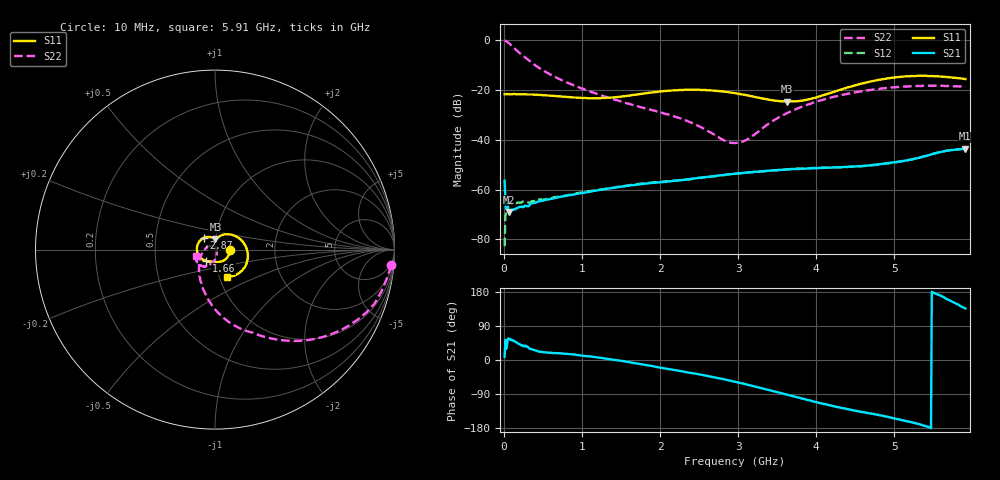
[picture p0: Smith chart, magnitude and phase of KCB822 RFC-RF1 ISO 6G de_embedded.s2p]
!Agilent	"Technologies,N5230A,MY45001650,A.07.50.48"
!Agilent	N5230A:	A.07.50.48
!Date:	"Wednesday,"	February	"12,"	2014	15:21:15
!Correction:	S11(Full	2	"Port(1,2))"
!S21(Full	2	"Port(1,2))"
!S12(Full	2	"Port(1,2))"
!S22(Full	2	"Port(1,2))"
!S2P	File:	Measurements:	"S11,"	"S21,"	"S12,"	S22:
#	Hz	S	dB	R	50
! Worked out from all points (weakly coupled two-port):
!   591 points, 10 MHz to 5.91 GHz, reference 50 ohm
!   highest |S21| = -43.60 dB at 5.9 GHz (marker M1); lowest = -69.0 dB at 60 MHz (marker M2)
!   lowest |S11| = -24.7 dB at 3.63 GHz (marker M3), VSWR 1.12, Z = 49.9 + j5.82 ohm
!   |S11| at or under -10 dB: start of sweep to end of sweep
!   |S22| runs from -41.3 to -0.1 dB; largest |S21 - S12| = 0.0016
!   S11 on the Smith chart (normalised r, x): 10 MHz: 1.18, -0.01; 1.66 GHz: 0.90, -0.12; 2.87 GHz: 0.87, +0.11; 5.91 GHz: 1.09, -0.34
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1e7  -21.70 -2.0  -56.40 8.3  -82.70 -164.0  -0.12 -5.2
4e7  -21.60 -3.9  -65.50 38.4  -65.30 10.4  -0.55 -18.8
6e7  -21.70 -5.3  -69.00 57.4  -63.80 34.0  -1.06 -26.2
8e7  -21.70 -6.9  -68.70 53.8  -65.20 115.0  -1.63 -33.0
1.1e8  -21.70 -9.6  -68.30 52.7  -65.80 -165.0  -2.53 -41.7
1.8e8  -21.70 -16.0  -67.30 44.1  -65.20 -85.6  -4.56 -57.1
3.5e8  -21.80 -31.9  -65.60 28.9  -64.90 27.8  -8.90 -86.2
5.6e8  -22.20 -51.2  -64.00 19.6  -63.70 21.6  -13.20 -109.0
1e9  -23.20 -85.9  -61.40 11.4  -61.10 13.1  -19.40 -143.0
1.66e9  -22.00 -127.0  -58.20 -7.6  -58.00 -8.0  -26.10 169.0
1.98e9  -20.70 -150.0  -57.10 -19.2  -56.90 -18.7  -28.80 147.0
2.38e9  -19.90 177.0  -55.80 -33.7  -55.80 -34.7  -32.90 121.0
2.87e9  -20.90 135.0  -53.90 -53.2  -53.90 -53.1  -40.80 52.1
2.96e9  -21.30 127.0  -53.60 -57.5  -53.70 -57.8  -41.30 27.7
3.13e9  -22.30 114.0  -53.10 -65.6  -53.10 -65.8  -39.60 -17.4
3.63e9  -24.70 87.7  -51.90 -91.7  -51.80 -91.7  -29.20 -74.8
3.95e9  -23.40 77.6  -51.40 -109.0  -51.30 -109.0  -25.20 -89.3
4.38e9  -19.20 51.5  -50.90 -129.0  -50.90 -129.0  -21.70 -104.0
4.93e9  -15.30 5.7  -49.30 -151.0  -49.40 -151.0  -19.10 -122.0
5.39e9  -14.30 -31.4  -46.60 -174.0  -46.60 -173.0  -18.30 -138.0
5.9e9  -15.60 -65.1  -43.60 137.0  -43.60 138.0  -18.70 -161.0
5.91e9  -15.60 -65.6  -43.60 136.0  -43.60 137.0  -18.80 -161.0
